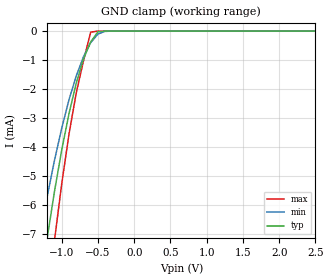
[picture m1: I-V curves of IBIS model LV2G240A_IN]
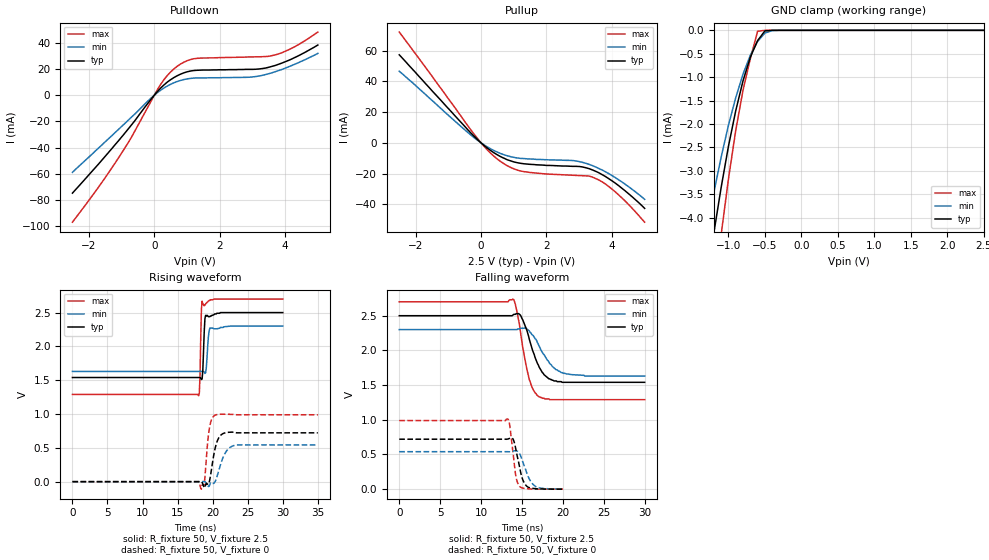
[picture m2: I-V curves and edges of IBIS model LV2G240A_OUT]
|/_/_/_/_/_/_/_/_/_/_/_/_/_/_/_/_/_/_/_/_/_/_/_/_/_/_/_/_/_/_/_/_/_/_/_/_/_/
|   Renesas Electronics Corp.
|   Multi Purpose Semiconductor Digital IC Design Group
|   IBIS Model of HD74LV2G240A
|   2.5V Dual Bus Buffer Inverted with 3-state Outputs,
|   SSOP-8(8pin) Package
|   History
|   V1.0   April   1, 2003   : First release.
|/_/_/_/_/_/_/_/_/_/_/_/_/_/_/_/_/_/_/_/_/_/_/_/_/_/_/_/_/_/_/_/_/_/_/_/_/_/
[IBIS Ver]   2.1
[Comment Char]  |_char
[File name]   l2g240s2.ibs
[File Rev]   1.1
[Date]   April 1, 2003
[Source]   Data created from SPICE simulations at
|   Renesas Electronics Corp.
[Notes]   RLC value of the Package is determined by assuming typical
|   conditions.
[Disclaimer]   This information is for modeling purposes only, and is not
|   guaranteed.
[Copyright]   Copyright 2003, Renesas Electronics Corp.,
|   All Rights Reserved.
|   Component  HD74LV2G240A
[Component]   HD74LV2G240A
[Manufacturer]  Renesas Electronics Corp.
[Package]
|   typ   min   max
R_pkg   0.099   0.095   0.102
L_pkg   1.740nH   1.680nH   1.790nH
C_pkg   0.140pF   0.140pF   0.150pF
[Pin]   signal_name   model_name   R_pin   L_pin   C_pin
1   G1   LV2G240A_IN   0.102   1.780nH   0.140pF
2   A1   LV2G240A_IN   0.097   1.710nH   0.150pF
3   Y2   LV2G240A_OUT   0.095   1.680nH   0.150pF
4   GND   GND   0.102   1.790nH   0.140pF
5   A2   LV2G240A_IN   0.101   1.790nH   0.140pF
6   Y1   LV2G240A_OUT   0.097   1.710nH   0.150pF
7   G2   LV2G240A_IN   0.097   1.710nH   0.150pF
8   VCC   POWER   0.102   1.790nH   0.140pF
| Models and submodels in the file (2): LV2G240A_IN (Input), LV2G240A_OUT (3-state)
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|   Model  LV2G240A_IN
[Model]   LV2G240A_IN
Model_type  Input
Vinl = 0.75V
Vinh = 1.75V
| variable   typ   min   max
C_comp   2.85pF   2.75pF   2.95pF
| variable   typ   min   max
[Temperature range]   25   85   -40
| variable   typ   min   max
[Voltage range]   2.5V   2.3V   2.7V
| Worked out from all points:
|   GND clamp passes 1 mA (typ) near -0.70 V on its own axis
[GND Clamp]
|   Voltage   I(typ)   I(min)   I(max)
-2.5V     -38.3mA    -30.7mA    -49.7mA
-1.3V     -8.88mA    -7.07mA    -11.7mA
-1.2V     -7.13mA    -5.7mA     -9.39mA
-1.1V     -5.53mA    -4.46mA    -7.22mA
-1V       -4.1mA     -3.35mA    -5.27mA
-900mV    -2.85mA    -2.37mA    -3.56mA
-800mV    -1.8mA     -1.55mA    -2.14mA
-700mV    -962uA     -887uA     -1.03mA
-600mV    -372uA     -399uA     -36.9uA
-500mV    -22uA      -101uA     -445nA
-400mV    -433nA     -10.3uA    -2.54nA
2.5V      5.09pA     27.7pA     5pA
|   Model  LV2G240A_OUT
[Model]   LV2G240A_OUT
Model_type  3-state
Polarity   Inverting
Enable   Active-Low
Vmeas = 1.25V
| variable   typ   min   max
C_comp   7.35pF   7.25pF   7.45pF
| variable   typ   min   max
[Temperature range]   25   85   -40
| variable   typ   min   max
[Voltage range]   2.5V   2.3V   2.7V
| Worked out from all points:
|   slope of the pulldown table from 0 to 0.375 V, typ, clamps not added: 39.2 ohm
|   slope of the pullup table from 0 to 0.375 V, typ, clamps not added: 60.8 ohm
|   GND clamp passes 1 mA (typ) near -0.78 V on its own axis
|   rising waveform, R_fixture 50, V_fixture 2.5: 20-80 % time 217ps typ, 271ps min, 172ps max; typ from 1.54 V to 2.5 V
|   rising waveform, R_fixture 50, V_fixture 0: 20-80 % time 801ps typ, 1.14ns min, 540ps max; typ from 0 V to 0.722 V
|   falling waveform, R_fixture 50, V_fixture 2.5: 20-80 % time 1.7ns typ, 2.12ns min, 1.31ns max; typ from 2.5 V to 1.54 V
|   falling waveform, R_fixture 50, V_fixture 0: 20-80 % time 825ps typ, 1.11ns min, 601ps max; typ from 0.72 V to 0 V
[Pullup]
|   Voltage   I(typ)   I(min)   I(max)
-2.5V     57.4mA     46.7mA     72.2mA
-200mV    4.01mA     3.18mA     5.31mA
200mV     -3.53mA    -2.75mA    -4.76mA
500mV     -7.83mA    -6.06mA    -10.6mA
900mV     -11.7mA    -8.98mA    -16mA
1.2V      -13.3mA    -10.1mA    -18.3mA
2.8V      -15.3mA    -11.5mA    -21.1mA
3.3V      -16.8mA    -14mA      -21.6mA
3.5V      -18.5mA    -15.7mA    -23.2mA
3.8V      -21.9mA    -18.8mA    -26.8mA
4.2V      -27.8mA    -24mA      -33.8mA
5V        -42.7mA    -36.8mA    -51.7mA
[Pulldown]
|   Voltage   I(typ)   I(min)   I(max)
-2.5V     -74.8mA    -58.9mA    -97mA
-1.6V     -49.6mA    -38mA      -66.6mA
-900mV    -29mA      -21.6mA    -40.4mA
200mV     5.59mA     3.93mA     8.44mA
400mV     10.1mA     7.08mA     15.1mA
700mV     14.9mA     10.5mA     22.1mA
1V        17.9mA     12.5mA     26.4mA
1.3V      19.1mA     13.3mA     28.2mA
2.9V      19.8mA     13.8mA     29.3mA
3.7V      22.8mA     18mA       30.9mA
4.3V      28.9mA     23.8mA     37.2mA
5V        38.4mA     32mA       48.3mA
[GND Clamp]
|   Voltage   I(typ)   I(min)   I(max)
-2.5V     -23.4mA    -18.8mA    -30.3mA
-1.3V     -5.4mA     -4.31mA    -7.13mA
-1.2V     -4.33mA    -3.47mA    -5.69mA
-1.1V     -3.36mA    -2.71mA    -4.37mA
-1V       -2.48mA    -2.03mA    -3.18mA
-900mV    -1.72mA    -1.44mA    -2.14mA
-800mV    -1.08mA    -936uA     -1.28mA
-700mV    -575uA     -533uA     -610uA
-600mV    -219uA     -237uA     -20.5uA
-500mV    -12.9uA    -58.6uA    -245nA
-400mV    -248nA     -6.13uA    -1.4nA
2.5V      2.62pA     30.9pA     2.5pA
[Ramp]
| variable   typ   min   max
dV/dt_r   0.433/800.9p   0.326/1.134n   0.593/539.6p
dV/dt_f   0.578/1.699n   0.400/2.122n   0.847/1.313n
R_load = 50ohms
[Rising Waveform]
R_fixture = 50
V_fixture = 2.5
V_fixture_min = 2.3
V_fixture_max = 2.7
C_fixture = 0p
|   Time   V(typ)   V(min)   V(max)
0s        1.54V      1.63V      1.29V
18ns      1.54V      1.63V      1.27V
18.1ns    1.54V      1.63V      1.31V
18.2ns    1.54V      1.63V      1.58V
18.4ns    1.51V      1.63V      2.55V
18.5ns    1.52V      1.63V      2.67V
18.9ns    2.41V      1.6V       2.61V
19ns      2.46V      1.61V      2.63V
19.6ns    2.44V      2.27V      2.68V
30ns      2.5V       2.3V       2.7V
[Rising Waveform]
R_fixture = 50
V_fixture = 0
C_fixture = 0p
|   Time   V(typ)   V(min)   V(max)
0s        -1.19uV    -3.47uV    112nV
18ns      -85.9uV    -34.7uV    1.89mV
18.4ns    2.75mV     -24.9uV    -111mV
18.8ns    -88.6mV    3.59mV     -39.3mV
19.4ns    -40.7mV    -71.7mV    690mV
19.8ns    158mV      -23.4mV    906mV
20.3ns    468mV      -9.47mV    980mV
21.7ns    720mV      407mV      997mV
23ns      732mV      533mV      994mV
35ns      722mV      543mV      989mV
[Falling Waveform]
R_fixture = 50
V_fixture = 2.5
V_fixture_min = 2.3
V_fixture_max = 2.7
C_fixture = 0p
|   Time   V(typ)   V(min)   V(max)
0s        2.5V       2.3V       2.7V
13.9ns    2.51V      2.3V       2.74V
14.3ns    2.53V      2.3V       2.61V
14.8ns    2.51V      2.32V      2.28V
15.3ns    2.38V      2.32V      1.91V
15.9ns    2.16V      2.28V      1.58V
17.1ns    1.76V      2.06V      1.33V
18.3ns    1.59V      1.83V      1.3V
19.8ns    1.55V      1.68V      1.29V
30ns      1.54V      1.63V      1.29V
[Falling Waveform]
R_fixture = 50
V_fixture = 0
C_fixture = 0p
|   Time   V(typ)   V(min)   V(max)
0s        720mV      540mV      989mV
13.3ns    723mV      540mV      1.01V
13.5ns    733mV      539mV      925mV
14ns      699mV      550mV      436mV
14.3ns    548mV      554mV      161mV
14.7ns    325mV      515mV      41.1mV
15ns      170mV      427mV      19.2mV
15.4ns    68.4mV     300mV      9.35mV
16.5ns    9.16mV     53.8mV     1.16mV
20ns      -2.72uV    -9.8uV     402nV
